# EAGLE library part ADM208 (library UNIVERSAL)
4x4 RS232 BUS TRANSCEIVER
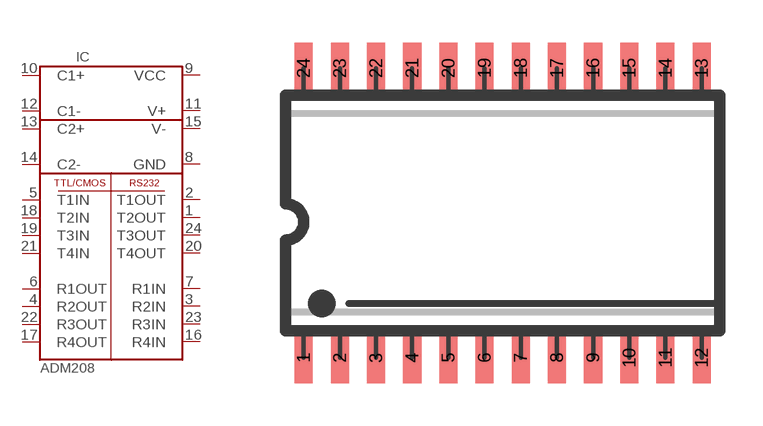
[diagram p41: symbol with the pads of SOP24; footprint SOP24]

Designator prefix IC

## ADM208 (IC: ADM208), ADM208ADM208  [SOP24]
1  T2OUT  out
2  T1OUT  out
3  R2IN  in
4  R2OUT  out
5  T1IN  in
6  R1OUT  out
7  R1IN  in
8  GND  pwr
9  VCC  pwr
10  C1+  pas
11  V+  pas
12  C1-  pas
13  C2+  pas
14  C2-  pas
15  V-  pas
16  R4IN  in
17  R4OUT  out
18  T2IN  in
19  T3IN  in
20  T4OUT  out
21  T4IN  in
22  R3OUT  out
23  R3IN  in
24  T3OUT  out

## Footprint SOP24 (pad centres in mm)
smd 0.635 x 1.778: 1 -5.715,-5.08; 2 -4.445,-5.08; 3 -3.175,-5.08; 4 -1.905,-5.08; 5 -0.635,-5.08; 6 0.635,-5.08; 7 1.905,-5.08; 8 3.175,-5.08; 9 4.445,-5.08; 10 5.715,-5.08; 11 6.985,-5.08; 12 8.255,-5.08; 13 8.255,5.08; 14 6.985,5.08; 15 5.715,5.08; 16 4.445,5.08; 17 3.175,5.08; 18 1.905,5.08; 19 0.635,5.08; 20 -0.635,5.08; 21 -1.905,5.08; 22 -3.175,5.08; 23 -4.445,5.08; 24 -5.715,5.08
